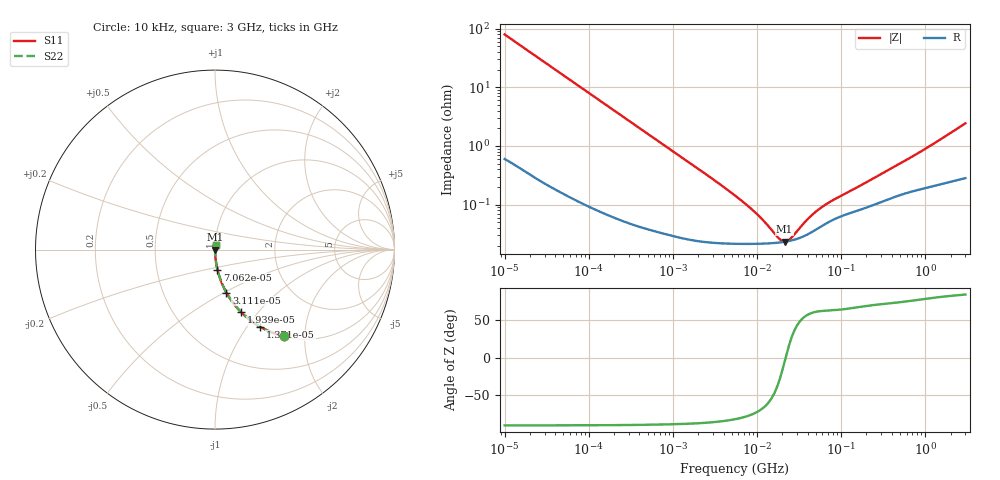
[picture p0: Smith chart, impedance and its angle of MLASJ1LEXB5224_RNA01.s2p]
! MLASJ1LEXB5224_RNA01  S-PARAMETER MODEL  ( Standard Model )
! Model Generated by TAIYO YUDEN Corporation (http://www.ty-top.com)
! Version 1.0
! TAIYO YUDEN Control No. 220601
! Copyright(c) 2015 TAIYO YUDEN CO.,LTD. All Rights Reserved.
! Product Description (link to TY-COMPAS)
! https://ds.yuden.co.jp/TYCOMPAS/or/detail?pn=MLASJ1LEXB5224KRNA01&u=M
! Products Name : Multilayer Ceramic Capacitors
! Characteristics :
!  Capacitance : 0.22 [uF] , Rated Voltage : 6.3 [V] , TCC : X5R
!  Case Size : 1.0 x 0.5 / 0.039 x 0.02 [mm/inch] , Thickness : 0.18 / 0.007 [mm/inch]
!  (Conditions: Temperature = 25 [degC] , DC Bias Voltage = 0 [V])
! External Node Assignments :
!  1  o---| |---o  2
! GND o---------o GND
! Frequency Range : 10kHz  -  3GHz  [ 401 STEP ]
# MHZ S RI R 50
! Freq[MHz].  S11 Real  S11 Imag  S21 Real  S21 Imag  S12 Real  S12 Imag  S22 Real  S22 Imag
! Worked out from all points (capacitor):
!   401 points, 10 kHz to 3 GHz, reference 50 ohm
!   read as one part in series: C = 200 nF near 10.65 kHz
!   lowest |Z| = 23.2 mohm at 21.25 MHz (marker M1)
!   series resonance near 21.91 MHz, so ESL is about 260 pH
!   S11 on the Smith chart (normalised r, x): 10 kHz: 1.01, -1.59; 13.71 kHz: 1.01, -1.16; 19.39 kHz: 1.01, -0.82; 31.11 kHz: 1.00, -0.51; 70.62 kHz: 1.00, -0.23; 3 GHz: 1.01, +0.05
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0.01  0.3872 -0.4834  0.6128 0.4834  0.6128 0.4834  0.3872 -0.4834
0.013707  0.2534 -0.431  0.7466 0.431  0.7466 0.431  0.2534 -0.431
0.019389  0.1464 -0.3494  0.8536 0.3494  0.8536 0.3494  0.1464 -0.3494
0.031113  0.0635 -0.2397  0.9365 0.2397  0.9365 0.2397  0.0635 -0.2397
0.070624  0.0138 -0.1118  0.9862 0.1118  0.9862 0.1118  0.0138 -0.1118
0.082683  0.0103 -0.0959  0.9897 0.0959  0.9897 0.0959  0.0103 -0.0959
0.199902  0.00222 -0.0402  0.9978 0.0402  0.9978 0.0402  0.00222 -0.0402
0.683653  0.000475 -0.0119  0.9995 0.0119  0.9995 0.0119  0.000475 -0.0119
5.477226  0.000216 -0.00141  0.9998 0.00141  0.9998 0.00141  0.000216 -0.00141
10.29003  0.000214 -0.000624  0.9998 0.000624  0.9998 0.000624  0.000214 -0.000624
18.15044  0.000224 -0.000143  0.9998 0.000143  0.9998 0.000143  0.000224 -0.000143
19.95104  0.000228 -7.06e-05  0.9998 7.06e-05  0.9998 7.06e-05  0.000228 -7.06e-05
21.24962  0.000231 -2.3e-05  0.9998 2.3e-05  0.9998 2.3e-05  0.000231 -2.3e-05
22.63272  0.000235 2.45e-05  0.9998 -2.45e-05  0.9998 -2.45e-05  0.000235 2.45e-05
24.87798  0.000241 9.59e-05  0.9998 -9.59e-05  0.9998 -9.59e-05  0.000241 9.59e-05
36.31858  0.000289 0.000391  0.9997 -0.000391  0.9997 -0.000391  0.000289 0.000391
45.28751  0.000341 0.000573  0.9997 -0.000573  0.9997 -0.000573  0.000341 0.000573
58.28018  0.000425 0.000784  0.9996 -0.000784  0.9996 -0.000784  0.000425 0.000784
75.00035  0.000523 0.000997  0.9995 -0.000997  0.9995 -0.000997  0.000523 0.000997
374.4521  0.00126 0.00375  0.9987 -0.00375  0.9987 -0.00375  0.00126 0.00375
905.3046  0.0019 0.00792  0.9981 -0.00792  0.9981 -0.00792  0.0019 0.00792
3000  0.00338 0.0239  0.9966 -0.0239  0.9966 -0.0239  0.00338 0.0239
